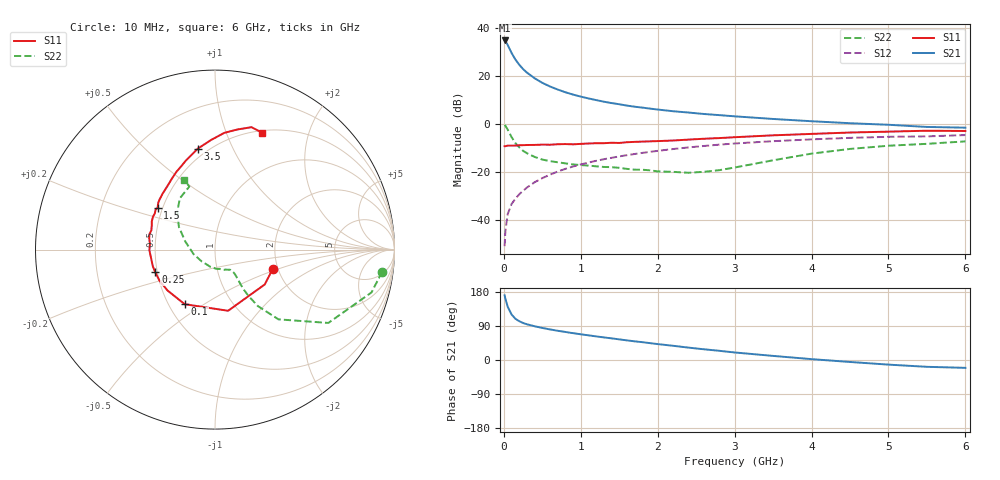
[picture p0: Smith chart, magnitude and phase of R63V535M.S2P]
! SIEMENS Small Signal Semiconductors
! BFR193
! Si NPN RF Bipolar Junction Transistor in SOT23
! VCE = 3.5 V  IC = 35 mA
! Common Emitter S-Parameters:  May  1996
# GHz  S  MA  R  50
!  f  S11  S21  S12  S22
! GHz  MAG  ANG  MAG  ANG  MAG  ANG  MAG  ANG
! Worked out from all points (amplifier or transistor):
!   36 points, 10 MHz to 6 GHz, reference 50 ohm
!   highest |S21| = 34.7 dB at 10 MHz (marker M1)
!   |S21| within 3 dB of that: start of sweep to 67.17 MHz
!   unconditionally stable (mu >= 1): 453.2 MHz to 2.002 GHz
!   at 250 MHz: K = 0.92, MSG = 25.4 dB, |S12| = -28.0 dB
!   at 1.4 GHz: K = 1.02, MAG = 10.6 dB, |S12| = -14.2 dB
!   at 6 GHz: K = 0.95, MSG = 1.5 dB, |S12| = -4.8 dB
!   S11 on the Smith chart (normalised r, x): 10 MHz: 1.88, -0.46; 100 MHz: 0.60, -0.42; 250 MHz: 0.49, -0.14; 1.5 GHz: 0.47, +0.26; 3.5 GHz: 0.44, +0.74; 6 GHz: 0.53, +1.35
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0.01  0.3393 -18.5  54.05 170.7  0.0028 85.0  0.9391 -7.6
0.02  0.3385 -35.0  52.43 161.8  0.0058 79.2  0.9041 -15.3
0.05  0.3486 -77.9  43.63 140.6  0.013 69.8  0.7523 -32.9
0.1  0.3479 -119.0  29.77 120.2  0.0211 67.0  0.5255 -47.7
0.15  0.349 -139.2  21.7 108.9  0.0272 66.9  0.3949 -52.8
0.2  0.3543 -150.5  16.9 102.4  0.0337 69.8  0.3207 -54.1
0.25  0.3559 -159.1  13.7 97.6  0.0399 70.6  0.2717 -54.3
0.3  0.3587 -165.1  11.57 94.3  0.0466 72.0  0.2418 -53.6
0.4  0.36 -173.6  8.818 89.1  0.0601 72.9  0.2026 -52.2
0.5  0.3656 -179.5  7.077 84.6  0.0733 72.9  0.1784 -51.0
0.6  0.3636 175.4  5.942 80.7  0.0865 72.4  0.1656 -50.9
0.7  0.3723 170.0  5.135 77.1  0.1005 71.6  0.1567 -51.5
0.8  0.3752 166.7  4.506 74.0  0.1142 70.7  0.1486 -52.4
0.9  0.3706 163.1  4.027 70.8  0.1279 69.7  0.1413 -52.9
1.1  0.3856 156.0  3.35 65.1  0.1545 67.6  0.1335 -57.3
1.5  0.3959 143.9  2.536 54.5  0.2074 62.1  0.12 -69.5
2.2  0.4452 125.9  1.813 37.5  0.2957 52.0  0.099 -106.3
3  0.521 108.3  1.42 19.9  0.3858 39.5  0.1219 -167.9
3.5  0.5705 99.7  1.251 10.8  0.4309 31.7  0.1723 164.5
4.5  0.6528 85.4  1.02 -5.2  0.5054 17.6  0.2972 135.0
5.5  0.7117 73.4  0.853 -18.0  0.5424 3.7  0.3795 112.1
6  0.7021 67.9  0.824 -20.7  0.5779 -0.4  0.4269 114.1
